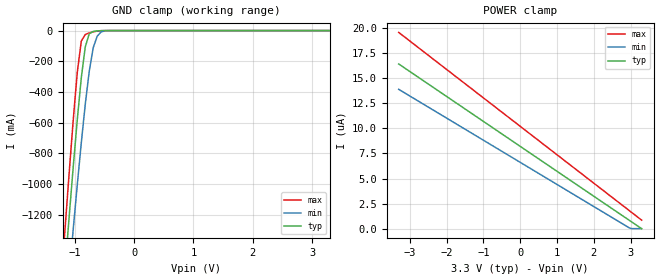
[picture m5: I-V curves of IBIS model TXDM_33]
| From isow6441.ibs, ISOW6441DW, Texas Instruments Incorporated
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|   TXDM_33 Model
[Model]   TXDM_33
Model_type Input
Polarity   Non-Inverting
Enable   Active-High
Vinl =  0.990V
Vinh =  2.310V
C_comp   1.300pF   1.100pF   1.500pF
[Model Spec]
Vinh   2.310V   2.079V   2.541V
Vinl   0.990V   0.891V   1.089V
[Temperature Range]   27.000   0.150k   -55.000
[Voltage Range]   3.300V   3.000V   3.600V
[POWER Clamp Reference]   3.300V   3.000V   3.600V
[GND Clamp Reference]   0.0V   0.0V   0.0V
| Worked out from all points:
|   GND clamp passes 1 mA (typ) near -0.58 V on its own axis
[GND_clamp]
|Voltage   I(typ)   I(min)   I(max)
-3.3V     -11.34A    -10.61A    -11.96A
-1.223V   -1.857A    -2.179A    -1.621A
-1.156V   -1.524A    -1.877A    -1.262A
-1.089V   -1.197A    -1.579A    -910.4mA
-1.022V   -879.3mA   -1.286A    -573.7mA
-955mV    -577.7mA   -1.002A    -269.8mA
-888mV    -307.2mA   -730.9mA   -68.38mA
-821mV    -105.6mA   -479.6mA   -25.34mA
-754mV    -20.65mA   -264.1mA   -15.58mA
-687mV    -5.628mA   -111.3mA   -8.153mA
-553mV    -520uA     -8.412mA   -685.9uA
3.3V      0A         0A         0A
[POWER_clamp]
|Voltage   I(typ)   I(min)   I(max)
-3.3V     16.43uA    13.9uA     19.57uA
2.965V    833.7nA    78.89nA    1.801uA
3.032V    667nA      0A         1.611uA
3.3V      0A         0A         851nA
